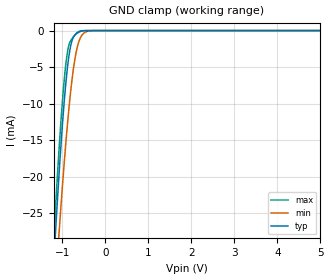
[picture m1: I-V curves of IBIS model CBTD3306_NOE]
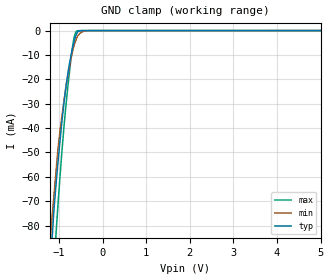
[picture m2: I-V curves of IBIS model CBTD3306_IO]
| TEXAS INSTRUMENTS INCORPORATED
| Standard Linear and Logic Group
| IBIS Model of SN74CBTD3306
| DUAL FET BUS SWITCH WITH LEVEL SHIFTING
| This file contains package information for the following:
|  TSSOP 8-pin (PW) package as [Component] CBTD3306_PW
|  SOIC 8-pin (D) package as [Component] CBTD3306_D
| This device can be powered at the following Vccs:
|  5 volt Vcc
| This file provides unique models under the [Model Selector] for each Vcc.
| For operation at a specific Vcc, select the appropriate model after each
| [Model Selector] keyword.
[IBIS Ver]   3.2
[Comment char]  |_char
[File Name]   sn74cbtd3306.ibs
[File Rev]   1.1 | a_die
[Date]   May 13, 2002
[Source]   Data created from TI-SPICE simulations at TI-SLL.
[Notes]   The following is an IBIS list for the CBTD3306.
   Please contact sllibis@ti.com with questions and
   comments concerning SLL IBIS models.
   This IBIS model is created from a BA (back annotated netlist
[Disclaimer] Property of Texas Instruments Incorporated.  Unauthorized
   reproduction and/or distribution is strictly prohibited.
   This product is protected under copyright law.
   Created  2002, (C) Copyright  2002, Texas Instruments
   Incorporated, All Rights Reserved
   UNLESS THERE IS A SIGNED, WRITTEN AGREEMENT TO THE
   CONTRARY, TEXAS INSTRUMENTS (TI) IS PROVIDING THE IBIS
   MODELS  AND WITHOUT ANY WARRANTY, EXPRESSED OR
   IMPLIED.  TI assumes no liability for:
   1) the accuracy of the IBIS models provided to your
   company;
   2) the proper functioning of these IBIS Models in your
   design or for any resulting applications; or
   3) infringement of patents, copyrights or intellectual
   property rights resulting from your use of these IBIS
   models.
   TI provides IBIS Models as a service to our customers.
   You and your company shall not distribute, sell or give
   these models to anyone else without prior written
   permission from TI.
   TI reserves the right to make changes to our products or
   to discontinue any semiconductor product or service
   without notice, and advises our customers to obtain the
   latest version of relevant information to verify, before
   placing orders, that the information being relied on is
   current.
   Please be aware that your receipt and use of the IBIS
   information provided shall serve as acceptance of these
   terms and conditions.  If you do not accept these terms,
   you should return or destroy the IBIS models and any
   other accompanying information immediately.
| Component CBTD3306_PW 8-pin TSSOP
[Component]   CBTD3306_PW
[Manufacturer]   Texas Instruments, Inc.
[Package]
|   typ   min   max
R_pkg   4.000e-02   3.400e-02   4.600e-02
L_pkg   2.625e-09   2.419e-09   2.861e-09
C_pkg   3.040e-13   2.860e-13   3.210e-13
[Pin]   signal_name   model_name   R_pin   L_pin   C_pin
1   1NOE   CBTD3306_NOE   4.600e-02   2.861e-09   3.210e-13
2   1A   CBTD3306_IO   3.700e-02   2.437e-09   2.860e-13
3   1B   CBTD3306_IO   3.400e-02   2.419e-09   2.860e-13
4   GND   GND   4.300e-02   2.784e-09   3.210e-13
5   2A   CBTD3306_IO   4.300e-02   2.784e-09   3.210e-13
6   2B   CBTD3306_IO   3.500e-02   2.420e-09   2.860e-13
7   2NOE   CBTD3306_NOE   3.700e-02   2.437e-09   2.860e-13
8   VCC   POWER   4.600e-02   2.860e-09   3.210e-13
| Component CBTD3306_D 8-pin SOIC
[Component]   CBTD3306_D
[Manufacturer]   Texas Instruments, Inc.
[Package]
|   typ   min   max
R_pkg   2.600e-02   1.700e-02   3.500e-02
L_pkg   2.637e-09   2.180e-09   3.093e-09
C_pkg   2.690e-13   2.240e-13   3.130e-13
[Pin]   signal_name   model_name   R_pin   L_pin   C_pin
1   1NOE   CBTD3306_NOE   3.500e-02   3.093e-09   3.130e-13
2   1A   CBTD3306_IO   1.700e-02   2.180e-09   2.240e-13
3   1B   CBTD3306_IO   1.700e-02   2.180e-09   2.240e-13
4   GND   GND   3.500e-02   3.093e-09   3.130e-13
5   2A   CBTD3306_IO   3.500e-02   3.093e-09   3.130e-13
6   2B   CBTD3306_IO   1.700e-02   2.180e-09   2.240e-13
7   2NOE   CBTD3306_NOE   1.700e-02   2.180e-09   2.240e-13
8   VCC   POWER   3.500e-02   3.093e-09   3.130e-13
[Series Switch Groups]
| Function Group States
On  1 /   | 1A->1B 1NOE,LOW
On  2 /   | 2A->2B 2NOE, LOW
On  1 2 /   | Enable Both
[Series Pin Mapping]   pin_2   model_name   function_table_group
2   3   CBTD3306_IO_50_S   1
5   6   CBTD3306_IO_50_S   2
[Model]   CBTD3306_IO_50_S
Model_type  Series_switch
| variable   typ   min   max
C_comp   0   0   0
[Temperature Range]   40   100   -40
| Ambient temperature   25   85   -40
[Voltage range]   5   4.5   5.5
[On]
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[Off]
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| Models and submodels in the file (3): CBTD3306_NOE (Input), CBTD3306_IO_50_S (Series_switch), CBTD3306_IO (Terminator)
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[Model]   CBTD3306_NOE
Model_type  Input
Vinl=0.8
Vinh=2.0
| variable   typ   min   max
C_comp   1.51pF   1.20pF   1.70pF
[Temperature Range]   40   100   -40
| Ambient temperature   25   85   -40
[Voltage range]   5   4.5   5.5
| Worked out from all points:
|   GND clamp passes 1 mA (typ) near -0.75 V on its own axis
[GND Clamp]
| CBTD3306_NOE_50
|   Voltage   I(typ)   I(min)   I(max)
-5V       -499.3mA   -428.8mA   -513.4mA
-1.185V   -30.81mA   -37.71mA   -27.5mA
-1.155V   -27.73mA   -35mA      -24.37mA
-1.06V    -18.58mA   -26.73mA   -15.19mA
-975mV    -11.46mA   -19.88mA   -8.326mA
-900mV    -6.364mA   -14.4mA    -3.922mA
-845mV    -3.604mA   -10.82mA   -2.038mA
-780mV    -1.57mA    -7.182mA   -1.182mA
-695mV    -558.9uA   -3.611mA   -543.9uA
-605mV    -200.3uA   -1.406mA   -101.8uA
-300mV    -29.91nA   -10.05uA   -1.516nA
5V        5.273nA    13.66nA    5.224nA
[Model]   CBTD3306_IO
Model_type  Terminator
| variable   typ   min   max
C_comp   3.30pF   2.77pF   3.81pF
| C_tri-state   3.30pF   2.77pF   3.81pF
[Temperature Range]   40   100   -40
| Ambient temperature   25   85   -40
[Voltage range]   5   4.5   5.5
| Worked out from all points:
|   GND clamp passes 1 mA (typ) near -0.59 V on its own axis
[GND Clamp]
| CBTD3306_IO_50
|   Voltage   I(typ)   I(min)   I(max)
-5V       -2.46A     -2.496A    -2.209A
-1.245V   -110.1mA   -95.5mA    -134.4mA
-1.18V    -91.53mA   -81.28mA   -115mA
-1.115V   -73.29mA   -67.42mA   -96.3mA
-1.065V   -62.5mA    -57.05mA   -82.54mA
-990mV    -47.65mA   -43.22mA   -63.09mA
-830mV    -21.68mA   -21.97mA   -28.75mA
-685mV    -6.871mA   -8.21mA    -6.097mA
-625mV    -2.809mA   -4.508mA   -1.085mA
-585mV    -954.4uA   -2.753mA   -106uA
-335mV    -204nA     -28.09uA   -7.276nA
5V        434.5pA    9.02nA     370.4pA
